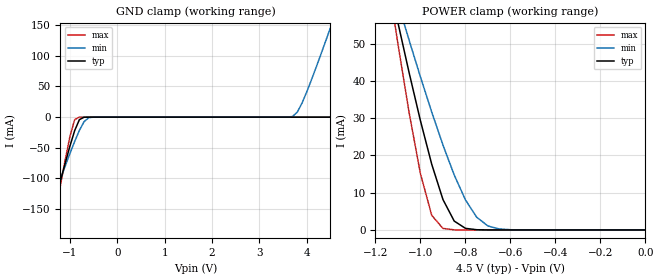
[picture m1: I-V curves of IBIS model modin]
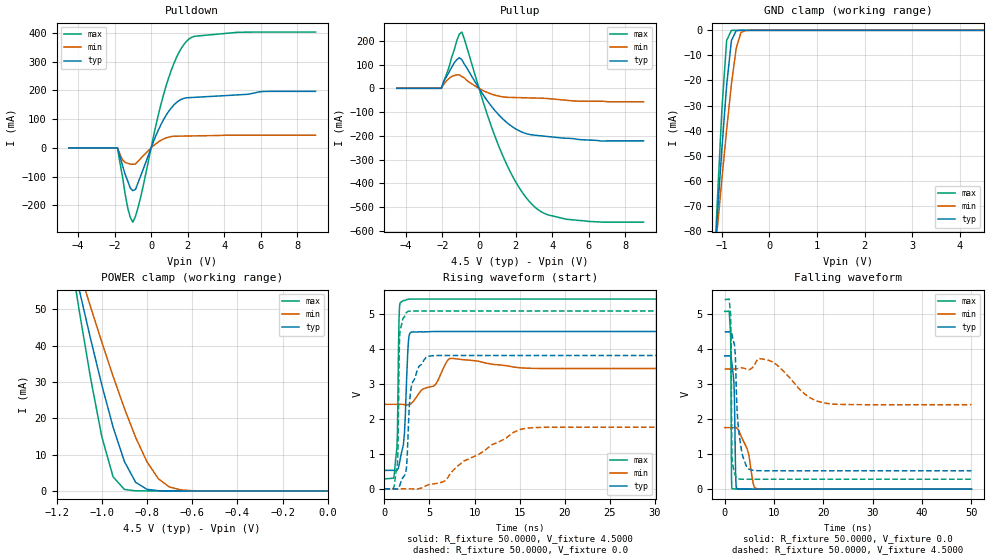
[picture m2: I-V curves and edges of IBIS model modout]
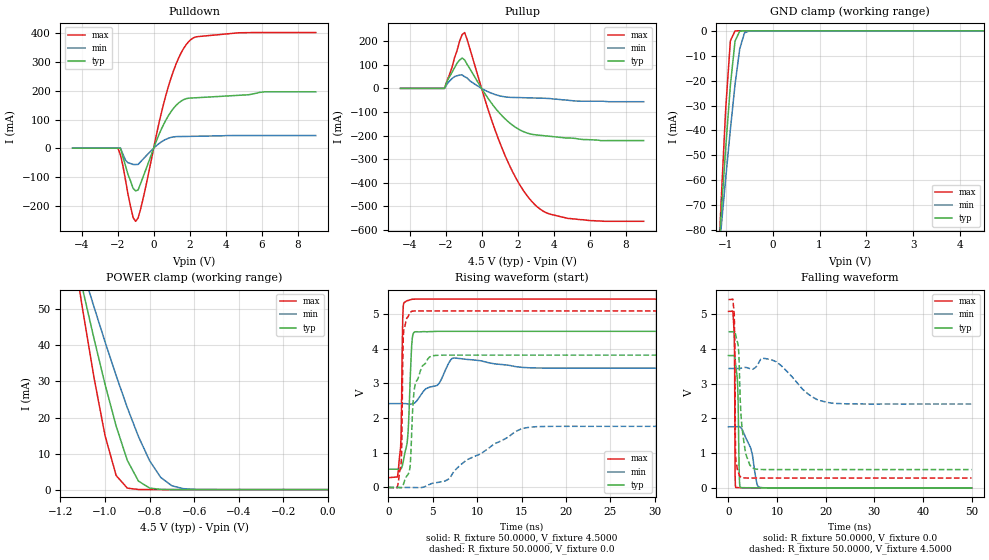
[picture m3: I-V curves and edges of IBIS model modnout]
| IBIS file 54ac74_pkg.ibs created by s2ibis3 verion 1.1
| North Carolina State University, ERL, 2006
[IBIS ver]  4.0
[File name] 54ac74_4v5_rev1.ibs
[File Rev]  1
[Date]   May 22 2009
[Source]   CAD & Design Solution (Catania) - STMicroelectronics
[Notes]
  (Note1) This IBIS model is the model of the product with package
   (Flat14 package elements);
  (Note2) This IBIS model is extracted with nominal 4.5V power supply
   (min:3.0V, typ:4.5V, max:5.5V);
  (Note3) This model has few Warnings about the non-monotonicity
   of I-V curves, but they are not indicative of problems
   inside the model;
[Copyright] (c) 2009 STMicroelectronics
|   Component 54AC74
[Component] 54AC74
[Manufacturer] STMicroelectronics
[Package]
| variable   typ   min   max
R_pkg   0.0   0.0   0.0
L_pkg   0.0H   0.0H   0.0H
C_pkg   0.0F   0.0F   0.0F
[Pin]   signal_name   model_name   R_pin   L_pin   C_pin
1   NCD1   modin   141.0m   4.31nH   1.01pF
2   D1   modin   108.1m   3.05nH   1.04pF
3   CP1   modin   90.5m   2.36nH   0.8pF
4   NSD1   modin   79.7m   1.96nH   0.8pF
5   Q1   modout   86.2m   2.16nH   0.8pF
6   NQ1   modnout   101.7m   2.85nH   1.04pF
7   GND   GND   111.0m   3.51nH   1.01pF
8   NQ2   modnout   141.0m   4.31nH   1.01pF
9   Q2   modout   112.4m   3.25nH   1.04pF
10   NSD2   modin   90.5m   2.36nH   0.8pF
11   CP2   modin   81.9m   2.06nH   0.8pF
12   D2   modin   84.0m   2.16nH   0.8pF
13   NCD2   modin   34.7m   0.86nH   0.80pF
14   VCC   POWER   111.0m   3.51nH   1.01pF
| Models and submodels in the file (3): modin (Input), modout (I/O), modnout (I/O)
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|   Model modin
[Model]   modin
Model_type Input
Vinl   =   1.35V
Vinh   =   3.15V
C_comp   0.532pF   NA   NA
[Temperature Range]   25.0000   0.1250k   -55.0000
[Voltage Range]   4.5000V   3.0000V   5.5000V
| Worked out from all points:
|   GND clamp passes 1 mA (typ) near -0.72 V on its own axis
|   POWER clamp passes 1 mA (typ) near -0.81 V on its own axis
[GND_clamp]
|Voltage   I(typ)   I(min)   I(max)
-4.5V     -1.124A    -840.2mA   -1.572A
-1.7V     -254mA     -209.8mA   -326.6mA
-1.6V     -223.6mA   -187.8mA   -282.8mA
-1.5V     -193.3mA   -165.8mA   -239.3mA
-1.4V     -163.2mA   -144mA     -196mA
-1V       -47.28mA   -59.41mA   -31.62mA
-900mV    -22mA      -39.68mA   -4.062mA
-800mV    -4.121mA   -21.58mA   -32.26uA
-500mV    -58.62nA   -53.9uA    -16.8pA
3.7V      5.8pA      1.071mA    3.8pA
3.9V      6.6pA      22.78mA    4.6pA
4.5V      9pA        145.6mA    7pA
[POWER_clamp]
|Voltage   I(typ)   I(min)   I(max)
-4.5V     1.102A     819.1mA    1.549A
-1.15V    69.49mA    71.07mA    69.5mA
-1.1V     55.56mA    60.84mA    49.84mA
-1.05V    42.07mA    50.81mA    31.3mA
-1V       29.27mA    41.04mA    15.03mA
-950mV    17.64mA    31.64mA    3.932mA
-900mV    8.156mA    22.78mA    419.2uA
-850mV    2.388mA    14.75mA    30.75uA
-800mV    435.6uA    8.064mA    2.159uA
-750mV    65.2uA     3.408mA    151.1nA
-700mV    9.379uA    1.071mA    10.58nA
0V        9pA        45.39pA    11pA
|   Model modout
[Model]  modout
Model_type I/O
Polarity Inverting
Vinl  =  1.35V
Vinh  =  3.15V
Vmeas =  2.25V
Cref  =  50pF
Rref  =  500
Vref  =  0
C_comp   2.7906pF   NA   NA
[Temperature Range]   25.0000   0.1250k   -55.0000
[Voltage Range]   4.5000V   3.0000V   5.5000V
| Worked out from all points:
|   slope of the pulldown table from 0 to 0.675 V, typ, clamps not added: 6.92 ohm
|   slope of the pullup table from 0 to 0.675 V, typ, clamps not added: 8.98 ohm
|   GND clamp passes 1 mA (typ) near -0.72 V on its own axis
|   POWER clamp passes 1 mA (typ) near -0.81 V on its own axis
|   rising waveform, R_fixture 50.0000, V_fixture 4.5000: 20-80 % time 428ps typ, 2.63ns min, 185ps max; typ from 0.527 V to 4.5 V
|   rising waveform, R_fixture 50.0000, V_fixture 0.0: 20-80 % time 646ps typ, 6.07ns min, 167ps max; typ from 0 V to 3.81 V
|   falling waveform, R_fixture 50.0000, V_fixture 0.0: 20-80 % time 307ps typ, 1.87ns min, 123ps max; typ from 3.81 V to 0 V
|   falling waveform, R_fixture 50.0000, V_fixture 4.5000: 20-80 % time 995ps typ, 4.4ns min, 158ps max; typ from 4.5 V to 0.527 V
[Pulldown]
|Voltage   I(typ)   I(min)   I(max)
-4.5V     0A         0A         0A
-1.84V    0A         0A         0A
-1.56V    -62mA      -42.13mA   -102mA
-1.28V    -114.9mA   -53.37mA   -208.7mA
-1V       -148.9mA   -56.95mA   -258.8mA
-580mV    -99.21mA   -37.58mA   -173.9mA
260mV     42.23mA    14.38mA    77.67mA
820mV     113.3mA    34.67mA    215.6mA
1.38V     157.3mA    40.54mA    313.4mA
1.94V     174.3mA    41.15mA    371.1mA
4.74V     184.4mA    44.04mA    402.3mA
9V        196.6mA    44.04mA    403mA
[Pullup]
|Voltage   I(typ)   I(min)   I(max)
-4.5V     0A         0A         0A
-2.06V    0A         0A         0A
-1.36V    106.9mA    53.37mA    160.7mA
-1.08V    128.9mA    56.95mA    227.8mA
-940mV    120.4mA    49.46mA    236.7mA
320mV     -37.87mA   -12.88mA   -79.72mA
1.16V     -118.1mA   -34.17mA   -258.5mA
2V        -170.6mA   -38.91mA   -393.2mA
2.84V     -195.4mA   -40.6mA    -483.8mA
3.54V     -201.3mA   -42.06mA   -525.6mA
4.8V      -210.4mA   -50.25mA   -551.6mA
9V        -221.4mA   -56.52mA   -563.7mA
[GND_clamp]
|Voltage   I(typ)   I(min)   I(max)
-4.5V     -1.124A    -840.2mA   -1.572A
-1.2V     -103.9mA   -101mA     -110.9mA
-1.1V     -75.04mA   -79.96mA   -69.91mA
-1V       -47.29mA   -59.4mA    -31.59mA
-900mV    -21.98mA   -39.67mA   -4.031mA
-800mV    -4.088mA   -21.54mA   -31.66uA
-700mV    -135.9uA   -7.225mA   -155.6nA
-600mV    -2.818uA   -878.4uA   -768.4pA
-500mV    -57.59nA   -52.91uA   -10.23pA
4.5V      72.03pA    374.6pA    144.1pA
[POWER_clamp]
|Voltage   I(typ)   I(min)   I(max)
-4.5V     1.102A     819.1mA    1.549A
-1.15V    69.46mA    71.06mA    69.48mA
-1.1V     55.53mA    60.83mA    49.81mA
-1.05V    42.04mA    50.8mA     31.27mA
-1V       29.24mA    41.03mA    15mA
-950mV    17.6mA     31.62mA    3.901mA
-900mV    8.117mA    22.74mA    412.3uA
-850mV    2.362mA    14.72mA    30.18uA
-800mV    428.4uA    8.027mA    2.118uA
-750mV    64uA       3.376mA    148.2nA
-700mV    9.203uA    1.058mA    10.38nA
0V        4.5pA      40.12pA    5.5pA
[Ramp]
| variable   typ   min   max
dV/dt_r  2.2883/0.7161n   1.0570/6.1505n   3.0521/0.8978n
dV/dt_f  2.3840/1.3013n   1.1659/8.7763n   3.0891/0.5394n
R_load = 50.0000
[Rising Waveform]
R_fixture= 50.0000
V_fixture= 4.5000
|time   V(typ)   V(min)   V(max)
0s        526.6mV    2.416V     283.7mV
1.14ns    525.4mV    2.416V     538mV
1.44ns    540.6mV    2.416V     1.581V
1.56ns    613.5mV    2.417V     4.008V
1.68ns    753mV      2.417V     5.239V
2.1ns     1.254V     2.412V     5.382V
2.64ns    4.145V     2.408V     5.422V
3ns       4.483V     2.445V     5.428V
7.44ns    4.5V       3.732V     5.428V
50ns      4.5V       3.44V      5.428V
[Rising Waveform]
R_fixture= 50.0000
V_fixture= 0.0
|time   V(typ)   V(min)   V(max)
0s        0V         0V         0V
1.38ns    -8.703mV   -14.82uV   587.5mV
1.5ns     633.1uV    -25.79uV   1.088V
1.68ns    83.44mV    -1.596uV   4.36V
2.4ns     523.4mV    206.8uV    5.028V
2.64ns    1.677V     -876.1uV   5.076V
3ns       2.944V     -2.952mV   5.086V
4.98ns    3.798V     122.6mV    5.087V
15.84ns   3.814V     1.734V     5.087V
50ns      3.814V     1.762V     5.087V
[Falling Waveform]
R_fixture= 50.0000
V_fixture= 0.0
|time   V(typ)   V(min)   V(max)
0s        3.814V     1.762V     5.087V
1.2ns     3.814V     1.762V     4.369V
1.26ns    3.794V     1.762V     3.762V
1.38ns    3.696V     1.761V     307mV
1.5ns     3.546V     1.762V     12.5mV
1.92ns    2.838V     1.764V     6.75mV
2.28ns    171.1mV    1.767V     6.661mV
2.7ns     4.866mV    1.712V     2.412mV
6.3ns     266uV      21.97mV    -6.171uV
50ns      2.691uV    1.329uV    2.567uV
[Falling Waveform]
R_fixture= 50.0000
V_fixture= 4.5000
|time   V(typ)   V(min)   V(max)
0s        4.5V       3.44V      5.428V
1.2ns     4.516V     3.44V      4.99V
1.32ns    4.496V     3.44V      4.052V
1.44ns    4.436V     3.44V      1.183V
1.5ns     4.401V     3.44V      850.8mV
2.04ns    4.062V     3.439V     442.4mV
2.46ns    2.421V     3.446V     316.5mV
3.66ns    942.8mV    3.468V     284.4mV
5.58ns    543.3mV    3.471V     283.7mV
50ns      526.6mV    2.416V     283.7mV
|   Model modnout
[Model]  modnout
Model_type I/O
Polarity Non-Inverting
Vinl  =  1.35V
Vinh  =  3.15V
Vmeas =  2.25V
Cref  =  50pF
Rref  =  500
Vref  =  0
C_comp   2.7906pF   NA   NA
[Temperature Range]   25.0000   0.1250k   -55.0000
[Voltage Range]   4.5000V   3.0000V   5.5000V
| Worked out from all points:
|   slope of the pulldown table from 0 to 0.675 V, typ, clamps not added: 6.92 ohm
|   slope of the pullup table from 0 to 0.675 V, typ, clamps not added: 8.98 ohm
|   GND clamp passes 1 mA (typ) near -0.72 V on its own axis
|   POWER clamp passes 1 mA (typ) near -0.81 V on its own axis
|   rising waveform, R_fixture 50.0000, V_fixture 4.5000: 20-80 % time 428ps typ, 2.63ns min, 185ps max; typ from 0.527 V to 4.5 V
|   rising waveform, R_fixture 50.0000, V_fixture 0.0: 20-80 % time 646ps typ, 6.07ns min, 167ps max; typ from 0 V to 3.81 V
|   falling waveform, R_fixture 50.0000, V_fixture 0.0: 20-80 % time 307ps typ, 1.87ns min, 123ps max; typ from 3.81 V to 0 V
|   falling waveform, R_fixture 50.0000, V_fixture 4.5000: 20-80 % time 995ps typ, 4.4ns min, 158ps max; typ from 4.5 V to 0.527 V
[Pulldown]
|Voltage   I(typ)   I(min)   I(max)
-4.5V     0A         0A         0A
-1.98V    0A         0A         0A
-1.84V    0A         0A         -24.21mA
-1.56V    -62mA      -42.13mA   -112mA
-1.14V    -140.1mA   -56.78mA   -242.1mA
-1V       -148.9mA   -56.95mA   -254.8mA
-720mV    -122.4mA   -46.99mA   -210.9mA
820mV     113.3mA    34.67mA    215.6mA
1.38V     157.3mA    40.54mA    313.4mA
1.94V     174.3mA    41.15mA    371.1mA
4.74V     184.4mA    44.04mA    402.3mA
9V        196.6mA    44.04mA    403mA
[Pullup]
|Voltage   I(typ)   I(min)   I(max)
-4.5V     0A         0A         0A
-2.06V    0A         0A         0A
-1.36V    106.9mA    53.37mA    160.7mA
-1.08V    128.9mA    56.95mA    227.8mA
-940mV    120.4mA    49.46mA    236.7mA
320mV     -37.87mA   -12.88mA   -79.72mA
1.16V     -118.1mA   -34.17mA   -258.5mA
2V        -170.6mA   -38.91mA   -393.2mA
2.84V     -195.4mA   -40.6mA    -483.8mA
3.54V     -201.3mA   -42.06mA   -525.6mA
4.8V      -210.4mA   -50.25mA   -551.6mA
9V        -221.4mA   -56.52mA   -563.7mA
[GND_clamp]
|Voltage   I(typ)   I(min)   I(max)
-4.5V     -1.124A    -840.2mA   -1.572A
-1.2V     -103.9mA   -101mA     -110.9mA
-1.1V     -75.04mA   -79.96mA   -69.91mA
-1V       -47.29mA   -59.4mA    -31.59mA
-900mV    -21.98mA   -39.67mA   -4.031mA
-800mV    -4.088mA   -21.54mA   -31.66uA
-700mV    -135.9uA   -7.225mA   -155.6nA
-600mV    -2.818uA   -878.4uA   -768.4pA
-500mV    -57.59nA   -52.91uA   -10.23pA
4.5V      72.03pA    374.6pA    144.1pA
[POWER_clamp]
|Voltage   I(typ)   I(min)   I(max)
-4.5V     1.102A     819.1mA    1.549A
-1.15V    69.46mA    71.06mA    69.48mA
-1.1V     55.53mA    60.83mA    49.81mA
-1.05V    42.04mA    50.8mA     31.27mA
-1V       29.24mA    41.03mA    15mA
-950mV    17.6mA     31.62mA    3.901mA
-900mV    8.117mA    22.74mA    412.3uA
-850mV    2.362mA    14.72mA    30.18uA
-800mV    428.4uA    8.027mA    2.118uA
-750mV    64uA       3.376mA    148.2nA
-700mV    9.203uA    1.058mA    10.38nA
0V        4.5pA      40.12pA    5.5pA
[Ramp]
| variable   typ   min   max
dV/dt_r  2.2883/0.7161n   1.0570/6.1505n   3.0521/0.8978n
dV/dt_f  2.3840/1.3013n   1.1659/8.7763n   3.0891/0.5394n
R_load = 50.0000
[Rising Waveform]
R_fixture= 50.0000
V_fixture= 4.5000
|time   V(typ)   V(min)   V(max)
0s        526.6mV    2.416V     283.7mV
1.14ns    525.4mV    2.416V     538mV
1.44ns    540.6mV    2.416V     1.581V
1.56ns    613.5mV    2.417V     4.008V
1.68ns    753mV      2.417V     5.239V
2.1ns     1.254V     2.412V     5.382V
2.64ns    4.145V     2.408V     5.422V
3ns       4.483V     2.445V     5.428V
7.44ns    4.5V       3.732V     5.428V
50ns      4.5V       3.44V      5.428V
[Rising Waveform]
R_fixture= 50.0000
V_fixture= 0.0
|time   V(typ)   V(min)   V(max)
0s        0V         0V         0V
1.38ns    -8.703mV   -14.82uV   587.5mV
1.5ns     633.1uV    -25.79uV   1.088V
1.68ns    83.44mV    -1.596uV   4.36V
2.4ns     523.4mV    206.8uV    5.028V
2.64ns    1.677V     -876.1uV   5.076V
3ns       2.944V     -2.952mV   5.086V
4.98ns    3.798V     122.6mV    5.087V
15.84ns   3.814V     1.734V     5.087V
50ns      3.814V     1.762V     5.087V
[Falling Waveform]
R_fixture= 50.0000
V_fixture= 0.0
|time   V(typ)   V(min)   V(max)
0s        3.814V     1.762V     5.087V
1.2ns     3.814V     1.762V     4.369V
1.26ns    3.794V     1.762V     3.762V
1.38ns    3.696V     1.761V     307mV
1.5ns     3.546V     1.762V     12.5mV
1.92ns    2.838V     1.764V     6.75mV
2.28ns    171.1mV    1.767V     6.661mV
2.7ns     4.866mV    1.712V     2.412mV
6.3ns     266uV      21.97mV    -6.171uV
50ns      2.691uV    1.329uV    2.567uV
[Falling Waveform]
R_fixture= 50.0000
V_fixture= 4.5000
|time   V(typ)   V(min)   V(max)
0s        4.5V       3.44V      5.428V
1.2ns     4.516V     3.44V      4.99V
1.32ns    4.496V     3.44V      4.052V
1.44ns    4.436V     3.44V      1.183V
1.5ns     4.401V     3.44V      850.8mV
2.04ns    4.062V     3.439V     442.4mV
2.46ns    2.421V     3.446V     316.5mV
3.66ns    942.8mV    3.468V     284.4mV
5.58ns    543.3mV    3.471V     283.7mV
50ns      526.6mV    2.416V     283.7mV
